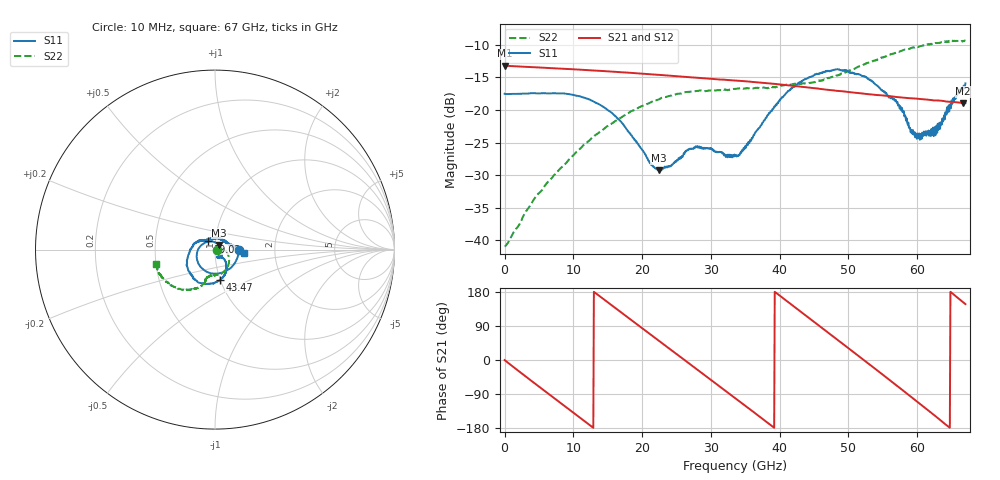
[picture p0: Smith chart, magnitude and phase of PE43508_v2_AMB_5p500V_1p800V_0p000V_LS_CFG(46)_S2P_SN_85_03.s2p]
!Keysight Technologies,N5227A,US51270237,A.10.43.00
!Date: Wednesday, August 22, 2018 17:11:22
!Correction: S11(Full 2 Port(1,3))
!S31(Full 2 Port(1,3))
!S13(Full 2 Port(1,3))
!S33(Full 2 Port(1,3))
!S2P File: Measurements: S11, S31, S13, S33:
# Hz S  dB  R 50
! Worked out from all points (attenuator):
!   801 points, 10 MHz to 67 GHz, reference 50 ohm
!   highest |S21| = -13.20 dB at 10 MHz (marker M1); lowest = -18.9 dB at 66.67 GHz (marker M2)
!   lowest |S11| = -29.3 dB at 22.45 GHz (marker M3), VSWR 1.07, Z = 52.3 + j2.65 ohm
!   |S11| at or under -10 dB: start of sweep to end of sweep
!   |S22| runs from -40.9 to -9.3 dB; largest |S21 - S12| = 0.001
!   S11 on the Smith chart (normalised r, x): 10 MHz: 1.31, -0.00; 19.02 GHz: 0.93, +0.08; 43.47 GHz: 1.00, -0.34; 67 GHz: 1.38, -0.05
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1e7  -17.51 -0.4  -13.20 -0.2  -13.20 -0.2  -40.88 -1.2
2.522125e9  -17.50 -30.6  -13.35 -35.8  -13.35 -35.8  -36.78 22.7
5.787888e9  -17.43 -67.8  -13.52 -81.1  -13.53 -81.1  -31.73 22.0
8.300012e9  -17.45 -96.3  -13.67 -115.7  -13.67 -115.7  -28.77 13.8
1.123082e10  -18.00 -128.6  -13.83 -156.0  -13.84 -155.9  -25.66 -0.9
1.47478e10  -19.80 -169.0  -14.06 155.8  -14.06 155.9  -22.65 -18.2
1.901841e10  -24.66 129.2  -14.36 97.4  -14.35 97.4  -19.96 -38.6
2.236791e10  -29.23 49.6  -14.61 51.7  -14.61 51.7  -18.38 -55.3
2.245165e10  -29.27 47.4  -14.62 50.5  -14.62 50.6  -18.38 -55.9
2.521499e10  -27.71 -16.6  -14.84 12.9  -14.84 12.9  -17.52 -68.0
2.797832e10  -25.69 -51.5  -15.06 -24.7  -15.06 -24.7  -17.10 -78.6
3.3505e10  -27.01 -65.1  -15.48 -100.2  -15.48 -100.2  -16.77 -93.8
3.852925e10  -20.42 -50.4  -15.92 -169.5  -15.92 -169.4  -16.51 -100.6
4.346976e10  -15.42 -79.8  -16.46 121.9  -16.45 121.9  -15.90 -105.2
4.472582e10  -14.84 -88.9  -16.60 104.4  -16.59 104.5  -15.80 -106.1
4.975008e10  -14.05 -126.7  -17.22 34.6  -17.21 34.6  -14.18 -107.8
5.251341e10  -14.97 -151.4  -17.53 -4.0  -17.51 -4.1  -12.86 -112.5
5.586291e10  -18.08 172.7  -17.85 -51.2  -17.84 -51.5  -11.56 -122.1
6.0301e10  -23.59 92.4  -18.30 -114.3  -18.30 -114.5  -10.27 -137.4
6.29806e10  -22.11 37.1  -18.53 -153.0  -18.55 -153.3  -9.74 -148.6
6.666505e10  -16.97 -3.5  -18.95 152.5  -19.00 152.6  -9.39 -164.2
6.7e10  -15.91 -6.2  -18.94 147.5  -19.00 147.5  -9.38 -166.4
